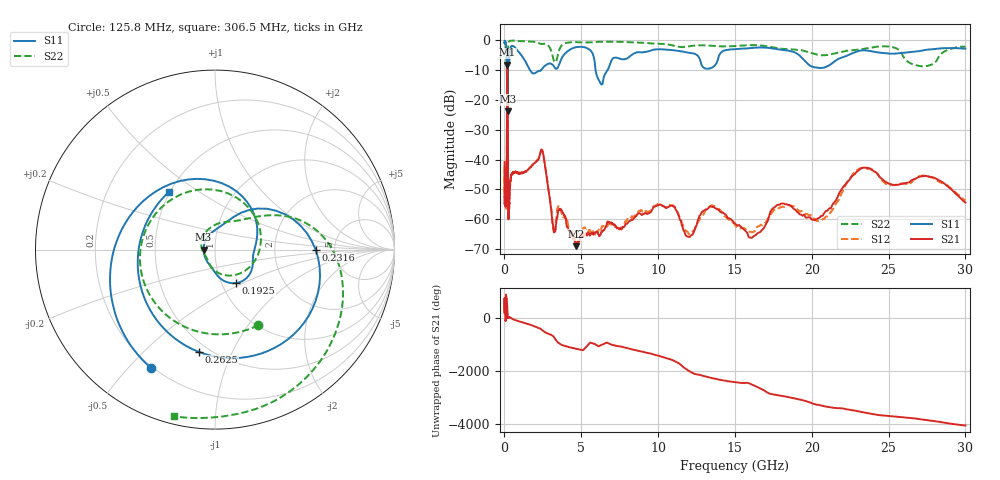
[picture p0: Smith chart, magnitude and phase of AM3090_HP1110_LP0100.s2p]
! Date/Time: Thu, Feb 28, 2019 2:08 PM
! Network Analyzer: Agilent Technologies E8364B Rev: A.07.50.67
! Sweep from 0.010 to 30.000 GHz, 1601 Points, Sweep Type: LOG
! Power Supply: 5.022 V, 0.002 A
# Hz S DB R 50
!freq MagS11 AngS11 MagS21 AngS21 MagS12 AngS12 MagS22 AngS22
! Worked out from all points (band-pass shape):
!   1601 points, 10 MHz to 30 GHz, reference 50 ohm
!   highest |S21| = -8.25 dB at 186.8 MHz (marker M1); lowest = -69.0 dB at 4.687 GHz (marker M2)
!   |S21| within 3 dB of the highest: 171.1 MHz to 205.5 MHz (34.35 MHz wide, 18.2 % of centre)
!   lowest |S11| = -23.9 dB at 207.5 MHz (marker M3), VSWR 1.14, Z = 44 - j0.104 ohm
!   |S11| at or under -10 dB: 165.1 MHz to 222.2 MHz (57.09 MHz wide, 29.5 % of centre); 1.649 GHz to 2.393 GHz (744.6 MHz wide, 36.8 % of centre); 5.931 GHz to 6.721 GHz (790.2 MHz wide, 12.5 % of centre)
!   |S22| runs from -23.9 to -0.2 dB; largest |S21 - S12| = 0.014
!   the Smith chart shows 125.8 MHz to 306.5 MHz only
!   S11 on the Smith chart (normalised r, x): 125.8 MHz: 0.19, -0.58; 192.5 MHz: 1.17, -0.46; 231.6 MHz: 3.55, +0.00; 262.5 MHz: 0.44, -0.75; 306.5 MHz: 0.49, +0.38
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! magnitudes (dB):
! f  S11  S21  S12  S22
! 10 MHz  -0.3  -40.9  -45.1  -0.6
! 38.04 MHz  -0.3  -50.4  -52.6  -1.1
! 125.8 MHz  -2.5  -50.2  -54.5  -6.3
! 144.7 MHz  -4.5  -49.0  -49.5  -7.8
! 166.5 MHz  -10.6  -14.8  -14.8  -15.0
! 186.8 MHz  -12.5  -8.3  -8.2  -22.4
! 192.5 MHz  -13.1  -8.5  -8.5  -19.5
! 207.5 MHz  -23.9  -12.3  -12.2  -12.6
! 231.6 MHz  -5.0  -44.7  -44.1  -2.5
! 262.5 MHz  -4.8  -59.9  -57.9  -0.8
! 306.5 MHz  -7.7  -56.2  -55.6  -0.4
! 550.5 MHz  -2.1  -44.2  -44.6  -0.2
! 2.084 GHz  -10.8  -40.6  -40.4  -0.8
! 2.47 GHz  -9.5  -37.0  -37.2  -1.3
! 3.204 GHz  -8.7  -64.0  -63.3  -6.7
! 4.687 GHz  -2.4  -69.0  -68.2  -0.7
! 6.234 GHz  -14.3  -65.3  -63.9  -0.6
! 7.926 GHz  -6.3  -61.5  -60.8  -0.7
! 16.29 GHz  -2.6  -65.5  -63.9  -1.7
! 20.82 GHz  -9.2  -57.9  -59.8  -5.1
! 23.48 GHz  -3.5  -42.7  -43.0  -2.9
! 30 GHz  -2.9  -54.4  -53.7  -2.2
